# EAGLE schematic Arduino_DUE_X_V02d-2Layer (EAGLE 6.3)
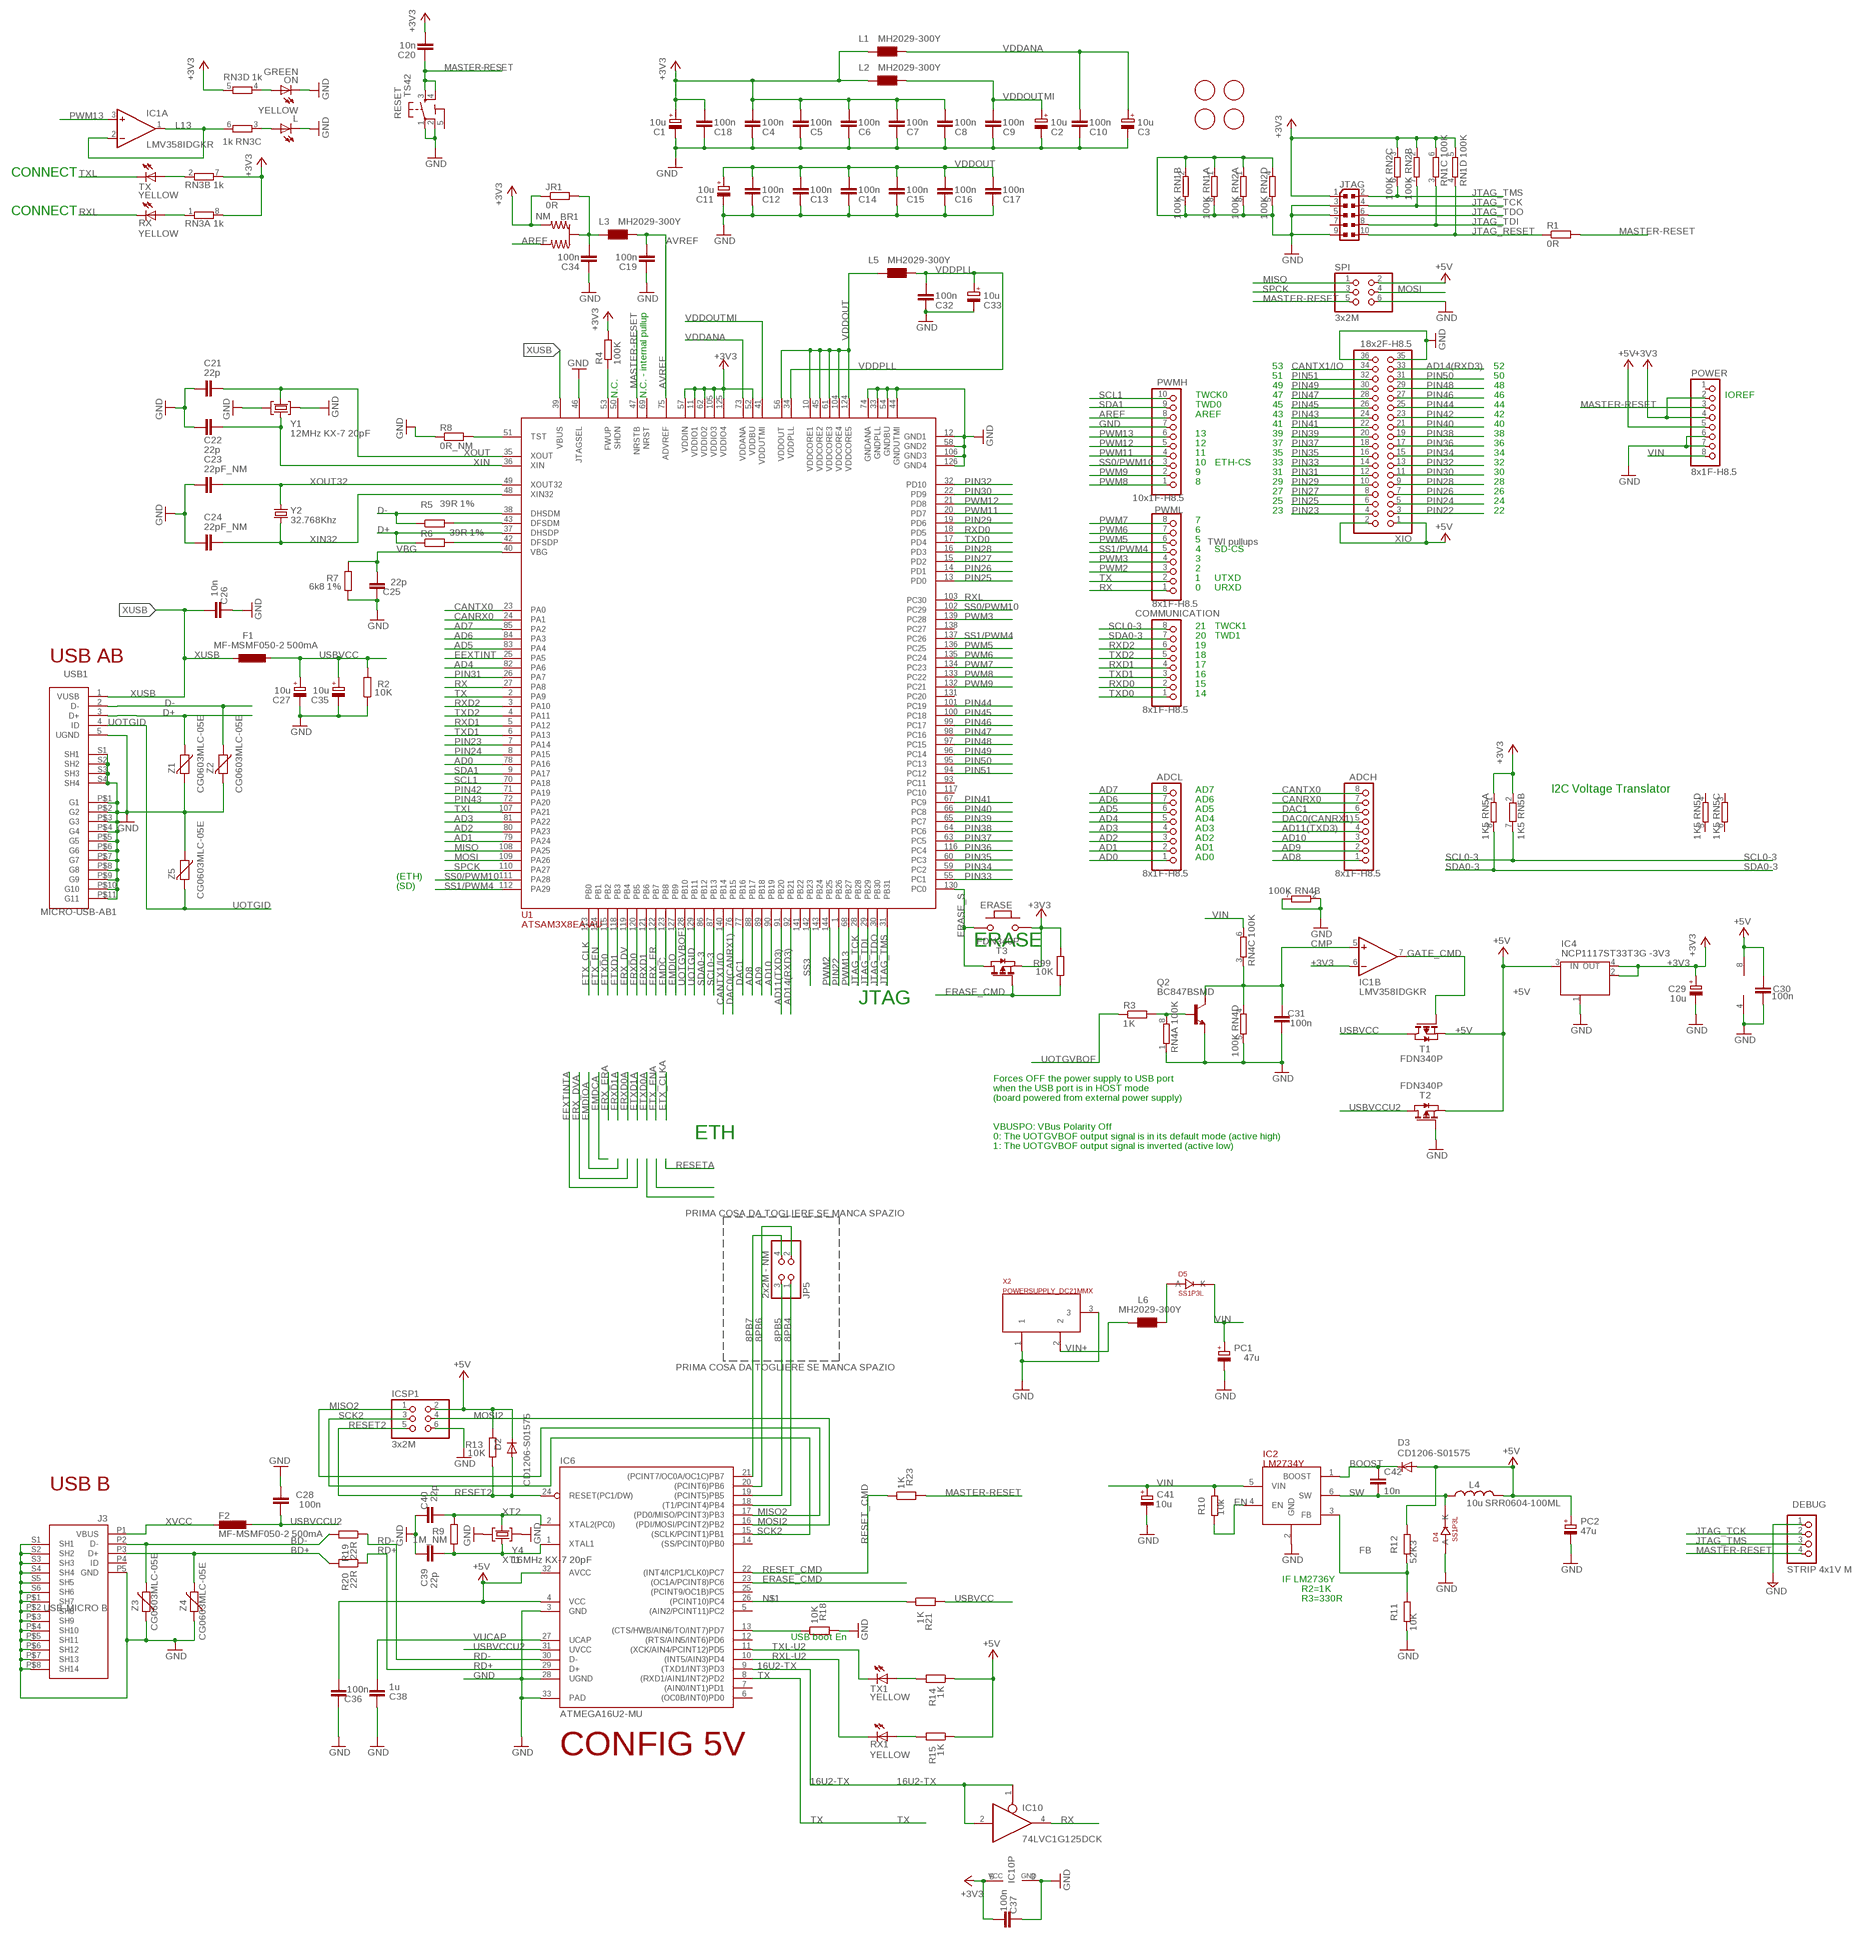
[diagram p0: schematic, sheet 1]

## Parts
ADCH  8x1F-H8.5  PINHD-1X8  [1X08]
ADCL  8x1F-H8.5  PINHD-1X8  [1X08]
BR1  NM  J0402  [J0402]
C1  10u  CPOL-EUSMCB  [SMC_B]
C2  10u  CPOL-EUSMCB  [SMC_B]
C3  10u  CPOL-EUSMCB  [SMC_B]
C4  100n  C-EUC0402  [C0402]
C5  100n  C-EUC0402  [C0402]
C6  100n  C-EUC0402  [C0402]
C7  100n  C-EUC0402  [C0402]
C8  100n  C-EUC0402  [C0402]
C9  100n  C-EUC0402  [C0402]
C10  100n  C-EUC0402  [C0402]
C11  10u  CPOL-EUSMCB  [SMC_B]
C12  100n  C-EUC0402  [C0402]
C13  100n  C-EUC0402  [C0402]
C14  100n  C-EUC0402  [C0402]
C15  100n  C-EUC0402  [C0402]
C16  100n  C-EUC0402  [C0402]
C17  100n  C-EUC0402  [C0402]
C18  100n  C-EUC0402  [C0402]
C19  100n  C-EUC0402  [C0402]
C20  10n  C-EUC0402  [C0402]
C21  22p  C-EUC0402  [C0402]
C22  22p  C-EUC0402  [C0402]
C23  22pF_NM  C-EUC0402  [C0402]
C24  22pF_NM  C-EUC0402  [C0402]
C25  22p  C-EUC0402  [C0402]
C26  10n  C-EUC0402  [C0402]
C27  10u  CPOL-EUSMCB  [SMC_B]
C28  100n  C-EUC0402  [C0402]
C29  10u  CPOL-EUSMCB  [SMC_B]
C30  100n  C-EUC0402  [C0402]
C31  100n  C-EUC0402  [C0402]
C32  100n  C-EUC0402  [C0402]
C33  10u  CPOL-EUSMCB  [SMC_B]
C34  100n  C-EUC0402  [C0402]
C35  10u  CPOL-EUSMCB  [SMC_B]
C36  100n  C-EUC0402  [C0402]
C37  100n  C-EUC0402  [C0402]
C38  1u  C-EUC0402  [C0402]
C39  22p  C-EUC0402  [C0402]
C40  22p  C-EUC0402  [C0402]
C41  10u  CPOL-EUSMCB  [SMC_B]
C42  10n  C-EUC0603  [C0603-ROUND]
COMMUNICATION  8x1F-H8.5  PINHD-1X8  [1X08]
D2  CD1206-S01575  DIODE-MINIMELF  [MINIMELF]
D3  CD1206-S01575  DIODE-MINIMELF  [MINIMELF]
D4  SS1P3L  [DO220AAL]
D5  SS1P3L  [DO220AAL]
DEBUG  STRIP 4x1V M  PINHD-1X4  [1X04]
ERASE  MYSMD_PB157  [SMD_157SW]
F1  MF-MSMF050-2 500mA  L-EUL1812  [L1812]
F2  MF-MSMF050-2 500mA  L-EUL1812  [L1812]
FID1  FIDUCIALMOUNT  [FIDUCIA-MOUNT]
FID2  FIDUCIALMOUNT  [FIDUCIA-MOUNT]
FID3  FIDUCIALMOUNT  [FIDUCIA-MOUNT]
FID4  FIDUCIALMOUNT  [FIDUCIA-MOUNT]
IC1  LMV358IDGKR  LMV358MMX  [MSOP08]
IC2  LM2734Y  LM2736Y  [SOT23-6]
IC4  NCP1117ST33T3G -3V3  MC33269ST-3.3T3  [SOT223]
IC6  ATMEGA16U2-MU  [MLF32]
IC10  74LVC1G125DCK  [SC70-5]
ICSP1  3x2M  PINHD-2X3  [2X03]
J3  USB-MICRO B  MYCON2_USB-MINI-B  [CON2_USB_MICRO_B_AT]
JP5  2x2M - NM  PINHD-2X2  [2X02]
JR1  0R  R-EU_R0402  [R0402]
JTAG  PINHEAD_PINHD-2X5PASSO127  [PINHEAD_2X05_127]
L  YELLOW  LEDCHIP-LED0805  [CHIP-LED0805]
L1  MH2029-300Y  WE-CBF_0805  [0805]
L2  MH2029-300Y  WE-CBF_0805  [0805]
L3  MH2029-300Y  WE-CBF_0805  [0805]
L4  10u SRR0604-100ML  L-USSRR0604  [SRR0604]
L5  MH2029-300Y  WE-CBF_0805  [0805]
L6  MH2029-300Y  WE-CBF_0805  [0805]
ON  GREEN  LEDCHIP-LED0805  [CHIP-LED0805]
PC1  47u  CPOL-EUD  [PANASONIC_D]
PC2  47u  CPOL-EUD  [PANASONIC_D]
POWER  8x1F-H8.5  PINHD-1X8  [1X08]
PWMH  10x1F-H8.5  PINHD-1X10  [1X10]
PWML  8x1F-H8.5  PINHD-1X8  [1X08]
Q2  BC847BSMD  [SOT23]
R1  0R  R-EU_R0402  [R0402]
R2  10K  R-EU_R0402  [R0402]
R3  1K  R-EU_R0402  [R0402]
R4  100K  R-EU_R0402  [R0402]
R5  39R 1%  R-EU_R0402  [R0402]
R6  39R 1%  R-EU_R0402  [R0402]
R7  6k8 1%  R-EU_R0603  [R0603-ROUND]
R8  0R_NM  R-EU_R0402  [R0402]
R9  1M_NM  R-EU_R0402  [R0402]
R10  10k  R-EU_R0402  [R0402]
R11  10K  R-EU_0603-RND  [R0603-ROUND]
R12  52K3  R-EU_0603-RND  [R0603-ROUND]
R13  10K  R-EU_R0402  [R0402]
R14  1K  R-EU_R0402  [R0402]
R15  1K  R-EU_R0402  [R0402]
R18  10K  R-EU_R0402  [R0402]
R19  22R  R-EU_R0402  [R0402]
R20  22R  R-EU_R0402  [R0402]
R21  1K  R-EU_R0402  [R0402]
R23  1K  R-EU_R0402  [R0402]
R99  10K  R-EU_R0402  [R0402]
RESET  TS42  [TS42]
RN1  100K  4R-NCAT16  [CAT16]
RN2  100K  4R-NCAT16  [CAT16]
RN3  1k  4R-NCAY16  [CAY16]
RN4  100K  4R-NCAT16  [CAT16]
RN5  1K5  4R-NCAT16  [CAT16]
RX  YELLOW  LEDCHIP-LED0805  [CHIP-LED0805]
RX1  YELLOW  LEDCHIP-LED0805  [CHIP-LED0805]
SPI  3x2M  PINHD-2X3  [2X03]
T1  FDN340P  PMOSSOT23  [SOT-23]
T2  FDN340P  PMOSSOT23  [SOT-23]
T3  FDN340P  PMOSSOT23  [SOT-23]
TX  YELLOW  LEDCHIP-LED0805  [CHIP-LED0805]
TX1  YELLOW  LEDCHIP-LED0805  [CHIP-LED0805]
U1  ATSAM3X8EA-AU  ATSAM3X/AAU  [LQFP144]
USB1  MICRO-USB-AB1  MICRO_USB  [MCR-AB1-S-RA-SMT]
X2  POWERSUPPLY_DC21MMX  [POWERSUPPLY_DC-21MM]
XIO  18x2F-H8.5  PINHD-2X18  [2X18]
Y1  12MHz KX-7 20pF  CRYSTAL-3.2-2.5  [CRYSTAL-3.2-2.5]
Y2  32.768Khz  RESONATOR_EPSON_FC_145  [RESONATOR_EPSON_FC_145]
Y4  16MHz KX-7 20pF  CRYSTAL-3.2-2.5  [CRYSTAL-3.2-2.5]
Z1  CG0603MLC-05E  VARISTORCN0603  [CT/CN0603]
Z2  CG0603MLC-05E  VARISTORCN0603  [CT/CN0603]
Z3  CG0603MLC-05E  VARISTORCN0603  [CT/CN0603]
Z4  CG0603MLC-05E  VARISTORCN0603  [CT/CN0603]
Z5  CG0603MLC-05E  VARISTORCN0603  [CT/CN0603]

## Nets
8PB4: IC6.18((T1/PCINT4)PB4) JP5.1
8PB5: IC6.19((PCINT5)PB5) JP5.3
8PB6: IC6.20((PCINT6)PB6) JP5.2
8PB7: IC6.21((PCINT7/OC0A/OC1C)PB7) JP5.4
16U2-TX: IC6.9((TXD1/INT3)PD3) IC10.1(OE) IC10.2(I)
+3V3: BR1.3 C1.+ C4.2 C5.2 C6.2 C7.2 C8.2 C18.2 C20.2 C29.+ C37.1 ERASE.1 IC1.6(B:-IN) IC4.2(OUT) IC4.4(OUT) IC10.5(VCC) JR1.1 JTAG.1 L1.1 L2.1 POWER.2 POWER.4 R4.2 R99.2 RN1.5 RN1.6 RN2.2 RN2.3 RN3.5 RN3.7 RN3.8 RN5.1 RN5.2 T3.2(S) U1.11(VDDIO1) U1.52(VDDBU) U1.57(VDDIN) U1.62(VDDIO2) U1.105(VDDIO3) U1.125(VDDIO4)
+5V: C30.2 C36.1 D2.C D3.A IC1.8(P:V+) IC4.3(IN) IC6.4(VCC) IC6.32(AVCC) ICSP1.2 L4.P$2 PC2.+ POWER.5 R12.1 R13.2 R14.1 R15.1 SPI.2 T1.2(S) T2.2(S) XIO.1 XIO.2
AD0: ADCL.1 U1.78(PA16)
AD1: ADCL.2 U1.79(PA24)
AD2: ADCL.3 U1.80(PA23)
AD3: ADCL.4 U1.81(PA22)
AD4: ADCL.5 U1.82(PA6)
AD5: ADCL.6 U1.83(PA4)
AD6: ADCL.7 U1.84(PA3)
AD7: ADCL.8 U1.85(PA2)
AD8: ADCH.1 U1.88(PB17)
AD9: ADCH.2 U1.89(PB18)
AD10: ADCH.3 U1.90(PB19)
AD11(TXD3): ADCH.4 U1.91(PB20)
AD14(RXD3): U1.92(PB21) XIO.33
AREF: BR1.1 PWMH.8
AVREF: C19.2 L3.2 U1.75(ADVREF)
AVREFL: BR1.2(C) C34.2 JR1.2 L3.1
BD+ [USB]: J3.P3(D+) R20.2 Z4.2
BD- [USB]: J3.P2(D-) R19.2 Z3.2
BOOST: C42.1 D3.C IC2.1(BOOST)
CANRX0: ADCH.7 U1.24(PA1)
CANTX0: ADCH.8 U1.23(PA0)
CANTX1/IO: U1.140(PB14) XIO.34
CMP: C31.2 IC1.5(B:+IN) Q2.3(C) RN4.3 RN4.4
D+ [USBpair]: R6.1 U1.37(DHSDP) USB1.3(D+) Z1.1
D- [USBpair]: R5.1 U1.38(DHSDM) USB1.2(D-) Z2.1
DAC0(CANRX1): ADCH.5 U1.76(PB15)
DAC1: ADCH.6 U1.77(PB16)
DTR: IC6.13((CTS/HWB/AIN6/TO/INT7)PD7) R18.1
EEXTINT: U1.25(PA5)
EMDC: U1.123(PB8)
EMDIO: U1.127(PB9)
EN: IC2.4(EN) R10.2
ERASE_CMD: IC6.23((OC1A/PCINT8)PC6) R99.1 T3.3(G)
ERASE_S: ERASE.2 T3.1(D) U1.130(PC0)
ERX_DV: U1.119(PB4)
ERX_ER: U1.122(PB7)
ERXD0: U1.120(PB5)
ERXD1: U1.121(PB6)
ETX_CLK: U1.113(PB0)
ETX_EN: U1.114(PB1)
ETXD0: U1.115(PB2)
ETXD1: U1.118(PB3)
FB: IC2.3(FB) R11.1 R12.2
GATE_CMD: IC1.7(B:OUT) T1.3(G)
GND: C1.- C2.- C3.- C4.1 C5.1 C6.1 C7.1 C8.1 C9.1 C10.1 C11.- C12.1 C13.1 C14.1 C15.1 C16.1 C17.1 C18.1 C19.1 C21.2 C22.2 C23.2 C24.2 C25.2 C26.2 C27.- C28.2 C29.- C30.1 C31.1 C32.1 C33.- C34.1 C35.- C36.2 C37.2 C38.2 C39.2 C40.2 C41.- D4.P$2(A) DEBUG.1 IC1.4(P:V-) IC2.2(GND) IC4.1(GND/ADJ) IC6.3(GND) IC6.28(UGND) IC6.33(PAD) IC10.3(GND) ICSP1.6 J3.P5(GND) J3.P$1(SH7) J3.P$2(SH8) J3.P$3(SH9) J3.P$4(SH10) J3.P$5(SH11) J3.P$6(SH12) J3.P$7(SH13) J3.P$8(SH14) J3.S1(SH1) J3.S2(SH2) J3.S3(SH3) J3.S4(SH4) J3.S5(SH5) J3.S6(SH6) JTAG.3 JTAG.5 JTAG.9 L.C ON.C PC1.- PC2.- POWER.6 POWER.7 PWMH.7 Q2.2(E) R2.1 R7.1 R8.1 R11.2 R18.2 RESET.1 RESET.2 RN1.1 RN1.2 RN1.7 RN1.8 RN2.1 RN2.4 RN2.5 RN2.8 RN4.1 RN4.2 RN4.5 RN4.7 SPI.6 T2.3(G) U1.12(GND1) U1.33(GNDPLL) U1.44(GNDUTMI) U1.46(JTAGSEL) U1.54(GNDBU) U1.58(GND2) U1.74(GNDANA) U1.106(GND3) U1.126(GND4) USB1.5(UGND) USB1.P$1(G1) USB1.P$2(G2) USB1.P$3(G3) USB1.P$4(G4) USB1.P$5(G5) USB1.P$6(G6) USB1.P$7(G7) USB1.P$8(G8) USB1.P$9(G9) USB1.P$10(G10) USB1.P$11(G11) USB1.S1(SH1) USB1.S2(SH2) USB1.S3(SH3) USB1.S4(SH4) X2.1 X2.3 XIO.35 XIO.36 Y1.2(GND) Y1.4(GND) Y4.2(GND) Y4.4(GND) Z1.2 Z2.2 Z3.1 Z4.1 Z5.1
JTAG_RESET: JTAG.10 R1.1 RN1.4
JTAG_TCK: DEBUG.2 JTAG.4 RN2.7 U1.28(PB28)
JTAG_TDI: JTAG.8 RN1.3 U1.29(PB29)
JTAG_TDO: JTAG.6 U1.30(PB30)
JTAG_TMS: DEBUG.3 JTAG.2 RN2.6 U1.31(PB31)
L13: IC1.1(A:OUT) IC1.2(A:-IN) RN3.6
MASTER-RESET: C20.1 DEBUG.4 POWER.3 R1.2 R23.2 RESET.3 RESET.4 SPI.5 U1.47(NRSTB)
MISO: SPI.1 U1.108(PA25)
MISO2: IC6.17((PD0/MISO/PCINT3)PB3) ICSP1.1
MOSI: SPI.4 U1.109(PA26)
MOSI2: IC6.16((PDI/MOSI/PCINT2)PB2) ICSP1.4
N$1: IC6.26((PCINT10)PC4) R21.1
N$2: L.A RN3.3
N$3: ON.A RN3.4
N$4: R15.2 RX1.A
N$5: R8.2 U1.51(TST)
N$6: Q2.1(B) R3.2 RN4.8
N$7: R4.1 U1.53(FWUP)
N$10: D5.P$2(A) L6.1
N$11: R5.2 U1.43(DFSDM)
N$12: R6.2 U1.42(DFSDP)
N$14: R14.2 TX1.A
N$54: RN3.1 RX.A
N$55: RN3.2 TX.A
PIN22: U1.1(PB26) XIO.3
PIN23: U1.7(PA14) XIO.4
PIN24: U1.8(PA15) XIO.5
PIN25: U1.13(PD0) XIO.6
PIN26: U1.14(PD1) XIO.7
PIN27: U1.15(PD2) XIO.8
PIN28: U1.16(PD3) XIO.9
PIN29: U1.19(PD6) XIO.10
PIN30: U1.22(PD9) XIO.11
PIN31: U1.26(PA7) XIO.12
PIN32: U1.32(PD10) XIO.13
PIN33: U1.55(PC1) XIO.14
PIN34: U1.59(PC2) XIO.15
PIN35: U1.60(PC3) XIO.16
PIN36: U1.116(PC4) XIO.17
PIN37: U1.63(PC5) XIO.18
PIN38: U1.64(PC6) XIO.19
PIN39: U1.65(PC7) XIO.20
PIN40: U1.66(PC8) XIO.21
PIN41: U1.67(PC9) XIO.22
PIN42: U1.71(PA19) XIO.23
PIN43: U1.72(PA20) XIO.24
PIN44: U1.101(PC19) XIO.25
PIN45: U1.100(PC18) XIO.26
PIN46: U1.99(PC17) XIO.27
PIN47: U1.98(PC16) XIO.28
PIN48: U1.97(PC15) XIO.29
PIN49: U1.96(PC14) XIO.30
PIN50: U1.95(PC13) XIO.31
PIN51: U1.94(PC12) XIO.32
PWM2: PWML.3 U1.144(PB25)
PWM3: PWML.4 U1.139(PC28)
PWM5: PWML.6 U1.136(PC25)
PWM6: PWML.7 U1.135(PC24)
PWM7: PWML.8 U1.134(PC23)
PWM8: PWMH.1 U1.133(PC22)
PWM9: PWMH.2 U1.132(PC21)
PWM11: PWMH.4 U1.20(PD7)
PWM12: PWMH.5 U1.21(PD8)
PWM13: IC1.3(A:+IN) PWMH.6 U1.68(PB27)
RD+: IC6.29(D+) R20.1
RD-: IC6.30(D-) R19.1
RESET2: D2.A IC6.24(RESET(PC1/DW)) ICSP1.5 R13.1
RESET_CMD: IC6.22((INT4/ICP1/CLK0)PC7) R23.1
RX: IC10.4(O) PWML.1 U1.27(PA8)
RXD0: COMMUNICATION.2 U1.18(PD5)
RXD1: COMMUNICATION.4 U1.5(PA12)
RXD2: COMMUNICATION.6 U1.3(PA10)
RXL: RX.C U1.103(PC30)
RXL-U2: IC6.10((INT5/AIN3)PD4) RX1.C
SCK2: IC6.15((SCLK/PCINT1)PB1) ICSP1.3
SCL0-3: COMMUNICATION.8 RN5.7 U1.87(PB13)
SCL1: PWMH.10 U1.70(PA18)
SDA0-3: COMMUNICATION.7 RN5.8 U1.86(PB12)
SDA1: PWMH.9 U1.9(PA17)
SPCK: SPI.3 U1.110(PA27)
SS0/PWM10: PWMH.3 U1.102(PC29) U1.111(PA28)
SS1/PWM4: PWML.5 U1.112(PA29) U1.137(PC26)
SS3: U1.142(PB23)
SW: C42.2 D4.P$1(K) IC2.6(SW) L4.P$1
TX: IC6.8((RXD1/AIN1/INT2)PD2) PWML.2 U1.2(PA9)
TXD0: COMMUNICATION.1 U1.17(PD4)
TXD1: COMMUNICATION.3 U1.6(PA13)
TXD2: COMMUNICATION.5 U1.4(PA11)
TXL: TX.C U1.107(PA21)
TXL-U2: IC6.11((XCK/AIN4/PCINT12)PD5) TX1.C
UOTGID: U1.129(PB11) USB1.4(ID) Z5.2
UOTGVBOF: R3.1 U1.128(PB10)
USBVCC: C27.+ C35.+ F1.1 R2.2 R21.2 T1.1(D)
USBVCCU2: C28.1 F2.1 IC6.31(UVCC) T2.1(D)
VBG: C25.1 R7.2 U1.40(VBG)
VDDANA: C3.+ C10.2 L1.2 U1.73(VDDANA)
VDDOUT: C11.+ C12.2 C13.2 C14.2 C15.2 C16.2 C17.2 L5.1 U1.10(VDDCORE1) U1.45(VDDCORE2) U1.56(VDDOUT) U1.61(VDDCORE3) U1.104(VDDCORE4) U1.124(VDDCORE5)
VDDOUTMI: C2.+ C9.2 L2.2 U1.41(VDDUTMI)
VDDPLL: C32.2 C33.+ L5.2 U1.34(VDDPLL)
VIN: C41.+ D5.P$1(K) IC2.5(VIN) PC1.+ POWER.8 R10.1 RN4.6
VIN+: L6.2 X2.2
VUCAP: C38.1 IC6.27(UCAP)
XIN: C22.1 U1.36(XIN) Y1.1(C1)
XIN32: C24.1 U1.48(XIN32) Y2.P$2
XOUT: C21.1 U1.35(XOUT) Y1.3(C2)
XOUT32: C23.1 U1.49(XOUT32) Y2.P$1
XT1: C39.1 IC6.1(XTAL1) R9.1 Y4.1(C1)
XT2: C40.1 IC6.2(XTAL2(PC0)) R9.2 Y4.3(C2)
XUSB [usbvcc]: C26.1 F1.2 U1.39(VBUS) USB1.1(VUSB)
XVCC [usbvcc]: F2.2 J3.P1(VBUS)
Unconnected: IC6.5((AIN2/PCINT11)PC2) IC6.6((OC0B/INT0)PD0) IC6.7((AIN0/INT1)PD1) IC6.12((RTS/AIN5/INT6)PD6) IC6.14((SS/PCINT0)PB0) IC6.25((PCINT9/OC1B)PC5) J3.P4(ID) JTAG.7 POWER.1 RN5.3 RN5.4 RN5.5 RN5.6 U1.50(SHDN) U1.69(NRST) U1.93(PC11) U1.117(PC10) U1.131(PC20) U1.138(PC27) U1.141(PB22) U1.143(PB24)

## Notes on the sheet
- CONNECT
- CONNECT
- 53 | 52
- 51 | 50
- 49 | 48
- N.C. | N.C. - internal pullup | TWCK0 | 47 | 46 | IOREF
- TWD0 | 45 | 44
- AREF | 43 | 42
- 41 | 40
- 13 | 39 | 38
- 12 | 37 | 36
- 11 | 35 | 34
- 10 | ETH-CS | 33 | 32
- 9 | 31 | 30
- 8 | 29 | 28
- 27 | 26
- 25 | 24
- 23 | 22
- 7
- 6
- 5 | TWI pullups
- 4 | SD-CS
- 3
- 2
- 1 | UTXD
- 0 | URXD
- 21 | TWCK1
- 20 | TWD1
- USB AB | 19
- 18
- 17
- 16
- 15
- 14
- AD7 | I2C Voltage Translator
- AD6
- AD5
- AD4
- AD3
- AD2
- AD1
- AD0
- (ETH)
- (SD)
- ERASE
- JTAG
- Forces OFF the power supply to USB port
- when the USB port is in HOST mode
- (board powered from external power supply)
- VBUSPO: VBus Polarity Off
- ETH | 0: The UOTGVBOF output signal is in its default mode (active high)
- 1: The UOTGVBOF output signal is inverted (active low)
- PRIMA COSA DA TOGLIERE SE MANCA SPAZIO
- PRIMA COSA DA TOGLIERE SE MANCA SPAZIO
- USB B
- IF LM2736Y
- R2=1K
- R3=330R
- USB boot En
- CONFIG 5V

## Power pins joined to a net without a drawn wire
5-GND: RESET.5(5-GND)

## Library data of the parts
ADCH ADCL COMMUNICATION POWER PWML = SmartPrj:PINHD-1X8: PIN HEADER
BR1 = bibaja:J: Three terminal jumper made from two 0402, 0603, 0805, etc.
C1-C3 C11 C27 C29 C33 C35 C41 PC1 PC2 = rcl:CPOL-EU: POLARIZED CAPACITOR, European symbol
C4-C10 C12-C26 C28 C30-C32 C34 C36-C40 C42 = SmartPrj:C-EU: CAPACITOR, European symbol
D2 D3 = diode:DIODE-: DIODE
D4 D5 = SmartPrj:SS1P3L
DEBUG = pinhead:PINHD-1X4: PIN HEADER
ERASE = SmartPrj:MYSMD_PB157
F1 F2 = rcl:L-EU: INDUCTOR, European symbol
FID1-FID4 = SmartPrj:FIDUCIALMOUNT
IC1 = linear:LMV358?*: Dual General Purpose, Low Voltage, Rail-to-Rail Output Operational Amplifiers Source: http://www.national.com/mpf/LM/LMV321.html http://www.national.com/dt/lmv_qual.pdf
IC2 = SmartPrj:LM2736Y
IC4 = linear:MC33269ST*: Adjustable Output Low Dropout Voltage Regulator 800 mA Source: http://www.onsemi.com/pub/Collateral/MC33269-D.PDF
IC6 = SmartPrj:ATMEGA16U2-
IC10 = 74xx-little-us:74*1G125: Single Bus Buffer Gate with 3-State Output
ICSP1 SPI = SmartPrj:PINHD-2X3: PIN HEADER
J3 = SmartPrj:MYCON2_USB-MINI-B
JP5 = SmartPrj:PINHD-2X2: PIN HEADER
JR1 R1-R15 R18-R21 R23 R99 = SmartPrj:R-EU_: RESISTOR, European symbol
JTAG = Arduino_Wifi_shield_v018_tG:PINHEAD_PINHD-2X5: PIN HEADER
L ON RX RX1 TX TX1 = led:LED: LED
L1-L3 L5 L6 = wuerth-elektronik:WE-CBF: SMD EMI Suppression Ferrite Beads
L4 = SmartPrj:L-US: INDUCTOR, American symbol
PWMH = SmartPrj:PINHD-1X10: PIN HEADER
Q2 = transistor-npn:BC847*: NPN Transistor
RESET = SmartPrj:TS42: TS42 Dongnan Electronics Tact switch VDC 12V - 50mA
RN1-RN5 = resistor-dil:4R-N: Array Chip Resistor Source: RS Component / Phycomp
T1-T3 = zetex:PMOSSOT23: MOS FET
U1 = SmartPrj:ATSAM3X/A
USB1 = SmartPrj:MICRO_USB: Micro_USB ADAM-TECH MCR-AB1-S-RA-SMT
X2 = SmartPrj:POWERSUPPLY_DC21MM
XIO = SmartPrj:PINHD-2X18: PIN HEADER
Y1 Y4 = SmartPrj:CRYSTAL-3.2-2.5
Y2 = Arduino_Wifi_shield_v018_tG:RESONATOR_EPSON_FC_145
Z1-Z5 = varistor:VARISTOR: VARISTOR

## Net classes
0 default: width 0.203 mm, drill 0.406 mm, clearance 0.203 mm
1 USB: width 0.203 mm, drill 0.406 mm, clearance 0.203 mm
2 gnd: width 0.203 mm, drill 0.406 mm, clearance 0.203 mm
3 usbvcc: width 0.203 mm, drill 0.406 mm, clearance 0.203 mm
4 USBpair: width 0.254 mm, drill 0.406 mm, clearance 0.61 mm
